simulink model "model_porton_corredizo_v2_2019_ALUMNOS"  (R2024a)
settings: Solver=ode45  StartTime=0.0  StopTime=100  MaxStep=.1  RelTol=1e-3
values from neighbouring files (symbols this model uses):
  c = 0    [Examen_Parcial_2_2026_ALUMNOS.m]
  m = 200    [Examen_Parcial_2_2026_ALUMNOS.m]
  magnitud_pulso_perturbacion = 100    [Examen_Parcial_2_2026_ALUMNOS.m]
  R = 0.05    [Examen_Parcial_2_2026_ALUMNOS.m]
  tiempo_pulso_perturbacion = 50    [Examen_Parcial_2_2026_ALUMNOS.m]
libraries: slpidlib x2

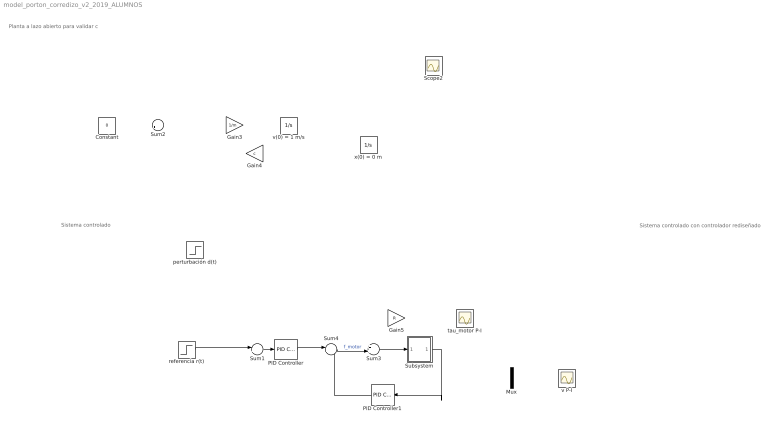
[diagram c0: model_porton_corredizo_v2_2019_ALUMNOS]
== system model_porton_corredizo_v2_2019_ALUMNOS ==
  note: Sistema controlado con controlador rediseñado
  note: Sistema controlado
  note: Planta a lazo abierto para validar c
  Constant : Constant  Value=0
  Gain3 : Gain  Gain=1/m
  Gain4 : Gain  Gain=c
  Gain5 : Gain  Gain=R
  Mux : Mux  Inputs=2
  PID Controller : slpidlib/PID Controller  Controller=PID  Form=Parallel  TimeDomain=Continuous-time  UseExternalTs=off  SampleTime=-1  IntegratorMethod=Forward Euler  FilterMethod=Forward Euler  ControllerParametersSource=internal  P=0  I=500  UseKiTs=off  D=0  UseExternalDerivativeSource=off  N=100  UseFilter=on  TunerSelectOption=Transfer Function Based (PID Tuner App)  InitialConditionSource=internal  InitialConditionForIntegrator=0  InitialConditionForFilter=0  DifferentiatorICPrevScaledInput=0  ExternalReset=none  TrackingMode=off  Kt=1  LimitOutput=off  SatLimitsSource=internal  UpperSaturationLimit=inf  LowerSaturationLimit=-inf  LinearizeAsGain=on  AntiWindupMode=none  Kb=1  LimitIntegrator=off  UpperIntegratorSaturationLimit=inf  LowerIntegratorSaturationLimit=-inf  POutMin=[]  POutMax=[]  IOutMin=[]  IOutMax=[]  DOutMin=[]  DOutMax=[]  NOutMin=[]  NOutMax=[]  SumOutMin=[]  SumOutMax=[]  SaturationOutMin=[]  SaturationOutMax=[]  PParamMin=[]  PParamMax=[]  IParamMin=[]  IParamMax=[]  DParamMin=[]  DParamMax=[]  NParamMin=[]  NParamMax=[]  KbParamMin=[]  KbParamMax=[]  KtParamMin=[]  KtParamMax=[]  KbOutMin=[]  KbOutMax=[]  KtOutMin=[]  KtOutMax=[]  IntegratorOutMin=[]  IntegratorOutMax=[]  FilterOutMin=[]  FilterOutMax=[]  SumI1OutMin=[]  SumI1OutMax=[]  SumI2OutMin=[]  SumI2OutMax=[]  SumI3OutMin=[]  SumI3OutMax=[]  SumI4OutMin=[]  SumI4OutMax=[]  SumDOutMin=[]  SumDOutMax=[]  DifferentiatorOutMin=[]  DifferentiatorOutMax=[]  FilterDiffOutCoefMin=[]  FilterDiffOutCoefMax=[]  ReciprocalOutMin=[]  ReciprocalOutMax=[]  SumDenOutMin=[]  SumDenOutMax=[]  SumNumOutMin=[]  SumNumOutMax=[]  DivideOutMin=[]  DivideOutMax=[]  UdiffTsProdOutMin=[]  UdiffTsProdOutMax=[]  NTsProdOutMin=[]  NTsProdOutMax=[]  UintegralTsProdOutMin=[]  UintegralTsProdOutMax=[]  UngainTsProdOutMin=[]  UngainTsProdOutMax=[]  ClampingZeroOutDataTypeStr=Inherit: Inherit via back propagation  ClampingZeroOutMin=[]  ClampingZeroOutMax=[]  FilterDenConstantOutDataTypeStr=Inherit: Inherit via back propagation  FilterDenConstantOutMin=[]  FilterDenConstantOutMax=[]  PCopyOutDataTypeStr=Inherit: Inherit via back propagation  PCopyOutMin=[]  PCopyOutMax=[]  NCopyOutDataTypeStr=Inherit: Inherit via back propagation  NCopyOutMin=[]  NCopyOutMax=[]  IntegratorContinuousStateAttributes=''  IntegratorStateMustResolveToSignalObject=off  IntegratorRTWStateStorageClass=Auto  FilterContinuousStateAttributes=''  FilterStateMustResolveToSignalObject=off  FilterRTWStateStorageClass=Auto  ParallelPVariant=InternalParameters  IdealPVariant=Disabled  IVariant=InternalParameters  DVariant=InternalParameters  IntegratorVariant=Continuous  SatVariant=Disabled  AWVariant=Passthrough  PCopyVariant=Disabled  TRVariant=Disabled  FdbkBlocksVariant=Forward  IdealPFdbkVariant=Disabled  SatFdbkVariant=Disabled  DerivativeFilterVariant=ContFilter  NVariant=InternalParameters  NCopyVariant=Disabled  FilterICVariant=InternalICsFilter  IntegratorICVariant=InternalICs  ExternalResetVariant=Disabled  TRSumVariant=Passthrough  SumFdbkVariant=Disabled  SumVariant=Sum_PID  TsampFilterVariant=InternalTs  TsampNgainVariant=Passthrough  TsampIntegralVariant=Disabled_SignalSpec  ExternalSaturationOutDataTypeStr=Inherit: Same as second input  DerivativeSourceVariant=ErrorSignal
  PID Controller1 : slpidlib/PID Controller  Controller=PID  Form=Parallel  TimeDomain=Continuous-time  UseExternalTs=off  SampleTime=-1  IntegratorMethod=Forward Euler  FilterMethod=Forward Euler  ControllerParametersSource=internal  P=2000  I=0  UseKiTs=off  D=0  UseExternalDerivativeSource=off  N=100  UseFilter=on  TunerSelectOption=Transfer Function Based (PID Tuner App)  InitialConditionSource=internal  InitialConditionForIntegrator=0  InitialConditionForFilter=0  DifferentiatorICPrevScaledInput=0  ExternalReset=none  TrackingMode=off  Kt=1  LimitOutput=off  SatLimitsSource=internal  UpperSaturationLimit=inf  LowerSaturationLimit=-inf  LinearizeAsGain=on  AntiWindupMode=none  Kb=1  LimitIntegrator=off  UpperIntegratorSaturationLimit=inf  LowerIntegratorSaturationLimit=-inf  POutMin=[]  POutMax=[]  IOutMin=[]  IOutMax=[]  DOutMin=[]  DOutMax=[]  NOutMin=[]  NOutMax=[]  SumOutMin=[]  SumOutMax=[]  SaturationOutMin=[]  SaturationOutMax=[]  PParamMin=[]  PParamMax=[]  IParamMin=[]  IParamMax=[]  DParamMin=[]  DParamMax=[]  NParamMin=[]  NParamMax=[]  KbParamMin=[]  KbParamMax=[]  KtParamMin=[]  KtParamMax=[]  KbOutMin=[]  KbOutMax=[]  KtOutMin=[]  KtOutMax=[]  IntegratorOutMin=[]  IntegratorOutMax=[]  FilterOutMin=[]  FilterOutMax=[]  SumI1OutMin=[]  SumI1OutMax=[]  SumI2OutMin=[]  SumI2OutMax=[]  SumI3OutMin=[]  SumI3OutMax=[]  SumI4OutMin=[]  SumI4OutMax=[]  SumDOutMin=[]  SumDOutMax=[]  DifferentiatorOutMin=[]  DifferentiatorOutMax=[]  FilterDiffOutCoefMin=[]  FilterDiffOutCoefMax=[]  ReciprocalOutMin=[]  ReciprocalOutMax=[]  SumDenOutMin=[]  SumDenOutMax=[]  SumNumOutMin=[]  SumNumOutMax=[]  DivideOutMin=[]  DivideOutMax=[]  UdiffTsProdOutMin=[]  UdiffTsProdOutMax=[]  NTsProdOutMin=[]  NTsProdOutMax=[]  UintegralTsProdOutMin=[]  UintegralTsProdOutMax=[]  UngainTsProdOutMin=[]  UngainTsProdOutMax=[]  ClampingZeroOutDataTypeStr=Inherit: Inherit via back propagation  ClampingZeroOutMin=[]  ClampingZeroOutMax=[]  FilterDenConstantOutDataTypeStr=Inherit: Inherit via back propagation  FilterDenConstantOutMin=[]  FilterDenConstantOutMax=[]  PCopyOutDataTypeStr=Inherit: Inherit via back propagation  PCopyOutMin=[]  PCopyOutMax=[]  NCopyOutDataTypeStr=Inherit: Inherit via back propagation  NCopyOutMin=[]  NCopyOutMax=[]  IntegratorContinuousStateAttributes=''  IntegratorStateMustResolveToSignalObject=off  IntegratorRTWStateStorageClass=Auto  FilterContinuousStateAttributes=''  FilterStateMustResolveToSignalObject=off  FilterRTWStateStorageClass=Auto  ParallelPVariant=InternalParameters  IdealPVariant=Disabled  IVariant=InternalParameters  DVariant=InternalParameters  IntegratorVariant=Continuous  SatVariant=Disabled  AWVariant=Passthrough  PCopyVariant=Disabled  TRVariant=Disabled  FdbkBlocksVariant=Forward  IdealPFdbkVariant=Disabled  SatFdbkVariant=Disabled  DerivativeFilterVariant=ContFilter  NVariant=InternalParameters  NCopyVariant=Disabled  FilterICVariant=InternalICsFilter  IntegratorICVariant=InternalICs  ExternalResetVariant=Disabled  TRSumVariant=Passthrough  SumFdbkVariant=Disabled  SumVariant=Sum_PID  TsampFilterVariant=InternalTs  TsampNgainVariant=Passthrough  TsampIntegralVariant=Disabled_SignalSpec  ExternalSaturationOutDataTypeStr=Inherit: Same as second input  DerivativeSourceVariant=ErrorSignal
  Scope2 : Scope
  Subsystem : Subsystem
  Sum1 : Sum  Inputs=|+-
  Sum2 : Sum  Inputs=|+-
  Sum3 : Sum  Inputs=++|
  Sum4 : Sum  Inputs=|+-
  perturbación d(t) : Step  Time=tiempo_pulso_perturbacion  After=-magnitud_pulso_perturbacion  SampleTime=0
  referencia r(t) : Step  SampleTime=0
  tau_motor P-I : Scope
  v P-I : Scope
  v(0) = 1 m/s : Integrator  InitialCondition=1
  x(0) = 0 m : Integrator  InitialCondition=1
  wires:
  Sum3/1 -> Subsystem/1(f)
  Sum4/1 -> Sum3/2  "f_motor"
  PID Controller1/1 -> Sum4/2
  PID Controller/1 -> Sum4/1
  Sum1/1 -> PID Controller/1
  referencia r(t)/1 -> Sum1/1
  Subsystem/1(v) -> PID Controller1/1

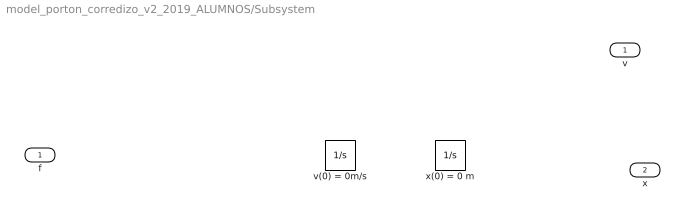
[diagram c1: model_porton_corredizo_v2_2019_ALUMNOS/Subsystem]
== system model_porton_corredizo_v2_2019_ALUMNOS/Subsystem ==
  f : Inport
  v(0) = 0m/s : Integrator
  x(0) = 0 m : Integrator
  v : Outport
  x : Outport  Port=2
